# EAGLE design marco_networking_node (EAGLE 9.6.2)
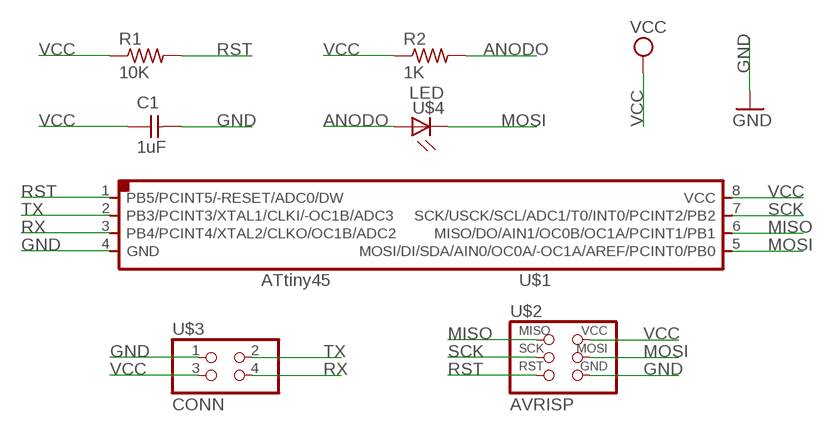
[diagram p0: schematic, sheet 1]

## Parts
C1  1uF  CAP_UNPOLARIZEDFAB  [C1206FAB]
R1  10K  R1206FAB  [R1206FAB]
R2  1K  R1206FAB  [R1206FAB]
U$1  ATTINY45  UC_ATTINY45SI  [SOIC8]
U$2  AVRISP  CONN_03X2_AVRISPSMD  [2X03SMD]
U$3  CONN  CONN_02X2-PINHEAD-SMD  [2X02SMD]
U$4  LED  LEDFAB1206  [LED1206FAB]

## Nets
ANODO: R2.2 U$4.1(A)
GND: C1.2 U$1.4(GND) U$2.6(GND) U$3.1
MISO: U$1.6(MISO/DO/AIN1/OC0B/OC1A/PCINT1/PB1) U$2.1(MISO)
MOSI: U$1.5(MOSI/DI/SDA/AIN0/OC0A/-OC1A/AREF/PCINT0/PB0) U$2.4(MOSI) U$4.2(C)
RST: R1.2 U$1.1(PB5/PCINT5/-RESET/ADC0/DW) U$2.5(RST)
RX: U$1.3(PB4/PCINT4/XTAL2/CLKO/OC1B/ADC2) U$3.4
SCK: U$1.7(SCK/USCK/SCL/ADC1/T0/INT0/PCINT2/PB2) U$2.3(SCK)
TX: U$1.2(PB3/PCINT3/XTAL1/CLKI/-OC1B/ADC3) U$3.2
VCC: C1.1 R1.1 R2.1 U$1.8(VCC) U$2.2(VCC) U$3.3

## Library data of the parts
C1 = fab:CAP_UNPOLARIZED
R1 R2 = fab:R: Resistor (US Symbol)
U$1 = fab:UC_ATTINY45
U$2 = fab:CONN_03X2_AVRISP
U$3 = fab:CONN_02X2-PINHEAD-SMD
U$4 = fab:LED: LED

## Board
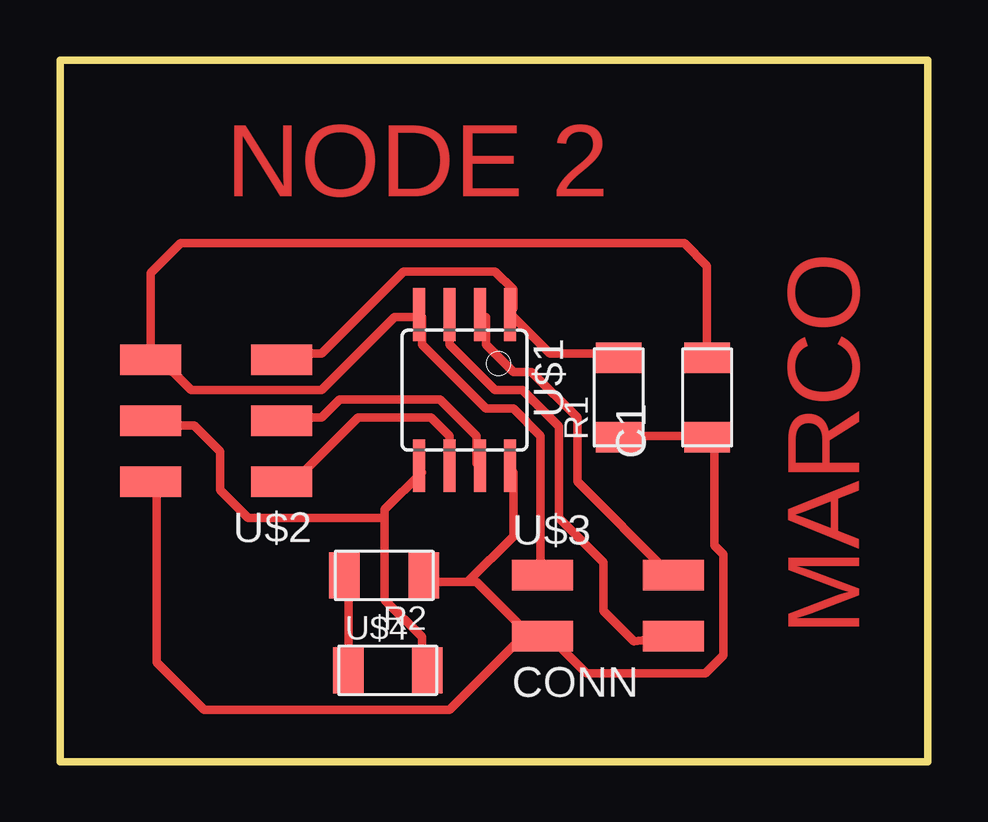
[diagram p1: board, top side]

Size 36.17 x 29.26 mm. Coordinates in mm from the lower left corner, seen from the top.
Outline: 0,29.26 36.17,29.26 36.17,0 0,0 0,29.26
Copper layers (1*16): Top 0.035mm / dielectric 1.5mm / Bottom 0.035mm
Design rules "fabcity-designrules *": minimum track width 14mil, minimum drill 32mil, track to track 16mil, track to pad 16mil, pad to pad 16mil, via to via 16mil, smd to smd 6mil, copper to edge 16mil, drill to drill 16mil, minimum pad ring 10mil, minimum via ring 8mil, stop-mask expansion 4mil, vias tented up to drill 0mil, thermal gap 16mil

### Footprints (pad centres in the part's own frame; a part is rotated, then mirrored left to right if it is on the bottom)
C1206FAB = smd 1.27 x 1.905: 1 -1.651,0; 2 1.651,0
R1206FAB = smd 1.27 x 1.905: 1 -1.651,0; 2 1.651,0
SOIC8 = smd 0.5 x 2.2: 1 -1.905,-3.154; 2 -0.645,-3.154; 3 0.625,-3.154; 4 1.895,-3.154; 5 1.905,3.154; 6 0.635,3.154; 7 -0.635,3.154; 8 -1.905,3.154
2X03SMD = smd 2.54 x 1.27: 1 -2.54,2.54; 2 2.92,2.54; 3 -2.54,0; 4 2.92,0; 5 -2.54,-2.54; 6 2.92,-2.54
2X02SMD = smd 2.54 x 1.27: 1 -2.54,1.27; 2 2.92,1.27; 3 -2.54,-1.27; 4 2.92,-1.27
LED1206FAB = smd 1.27 x 1.905: 1 -1.651,0; 2 1.651,0

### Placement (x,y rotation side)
C1  26.97,15.19 90 top
R1  23.29,15.19 90 top
R2  13.51,7.77 180 top
U$1  16.87,15.49 180 top
U$2  6.71,14.22 180 top
U$3  22.66,6.5 0 top
U$4  13.67,3.81 0 top

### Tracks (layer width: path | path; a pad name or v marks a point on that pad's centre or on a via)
ANODO
  Top 0.356: R2.2 12.04,7.49 12.04,4.06 U$4.1
GND
  Top 0.356: C1.2 26.97,20.68 26.03,21.61 5.03,21.61 3.79,20.37 U$2.6 4.04,17.02 4.04,16.92 5.46,15.49 10.9,15.49 13.94,18.54 15.09,18.54 | 15.09,18.54 15.09,17.4 17.75,14.73 18.9,14.73 20.04,13.59 20.04,7.87 U$3.1 | 15.09,18.54 U$1.4
MISO
  Top 0.356: U$1.6 16.23,13.59 15.47,14.35 12.42,14.35 9.75,11.68 U$2.1
MOSI
  Top 0.356: 13.54,10.16 13.54,10.52 15.09,12.07 U$1.5 | 13.54,10.16 13.54,6.76 15.09,5.21 15.09,4.06 U$4.2 | 13.54,10.16 7.85,10.16 6.68,11.33 6.68,12.93 5.59,14.02 4.09,14.02 4.04,13.97 U$2.4
RST
  Top 0.356: R1.2 23.09,17.02 20.42,17.02 18.9,18.54 U$1.1 18.9,18.92 18.9,19.68 18.14,20.45 14.33,20.45 10.9,17.02 9.37,17.02 U$2.5
RX
  Top 0.356: U$1.3 16.23,18.54 16.23,17.4 18.14,15.49 19.28,15.49 20.8,13.97 20.8,10.16 22.66,8.31 22.66,6.3 23.93,5.03 U$3.4
SCK
  Top 0.356: U$1.7 17.37,12.45 17.37,13.59 15.85,15.11 11.66,15.11 10.9,14.35 9.37,14.35 U$2.3
TX
  Top 0.356: U$1.2 17.75,18.54 17.75,17.4 18.9,16.26 19.66,16.26 21.56,14.35 21.56,11.68 25.37,7.87 U$3.2
VCC
  Top 0.356: R1.1 23.47,13.59 26.9,13.59 C1.1 27.28,13.21 27.28,9.02 27.66,8.64 27.66,4.45 26.9,3.68 21.95,3.68 20.42,5.21 U$3.3 | 16.99,7.49 17.37,7.49 19.28,5.59 19.66,5.59 | 16.99,7.49 15.47,7.49 R2.1 | 19.66,5.59 20.04,5.59 U$3.3 | 16.99,7.49 18.9,9.4 18.9,12.07 U$1.8 | 19.66,5.59 16.23,2.16 6.02,2.16 4.04,4.14 4.04,11.68 U$2.2 | 19.66,5.59 U$3.3

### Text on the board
Top: NODE 2 | MARCO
